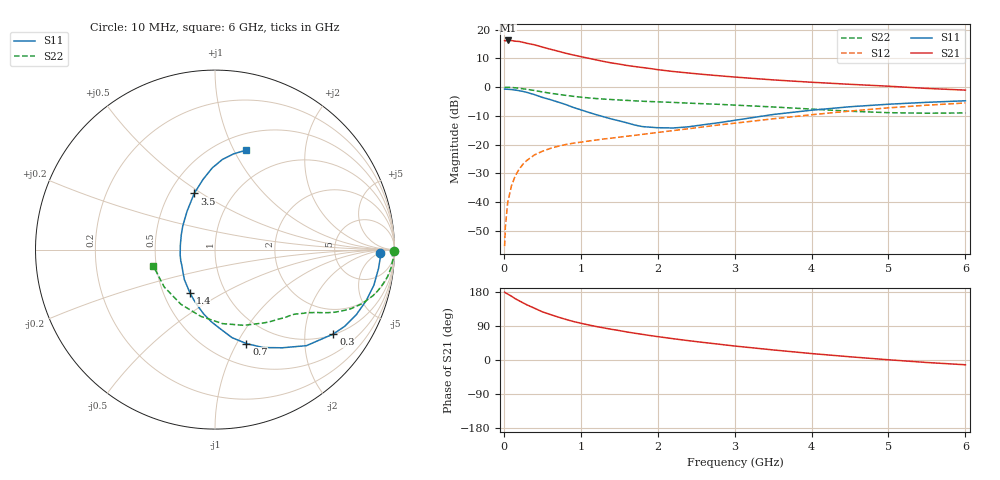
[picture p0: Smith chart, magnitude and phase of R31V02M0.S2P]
! SIEMENS Small Signal Semiconductors
! BFR181
! Si NPN RF Bipolar Junction Transistor in SOT23
! VCE = 1 V  IC = 2 mA
! Common Emitter S-Parameters:  May  1996
# GHz  S  MA  R  50
!  f  S11  S21  S12  S22
! GHz  MAG  ANG  MAG  ANG  MAG  ANG  MAG  ANG
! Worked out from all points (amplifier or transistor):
!   36 points, 10 MHz to 6 GHz, reference 50 ohm
!   highest |S21| = 16.3 dB at 50 MHz (marker M1)
!   |S21| within 3 dB of that: start of sweep to 597.3 MHz
!   unconditionally stable (mu >= 1): 1.503 GHz to 3.56 GHz
!   at 250 MHz: K = 0.24, MSG = 21.2 dB, |S12| = -26.8 dB
!   at 1.4 GHz: K = 0.97, MSG = 13.1 dB, |S12| = -17.8 dB
!   at 6 GHz: K = 0.89, MSG = 2.2 dB, |S12| = -5.5 dB
!   S11 on the Smith chart (normalised r, x): 10 MHz: 23, -6; 300 MHz: 1.02, -2.79; 700 MHz: 0.73, -1.10; 1.4 GHz: 0.68, -0.35; 3.5 GHz: 0.66, +0.47; 6 GHz: 0.67, +1.11
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0.01  0.922 -1.3  6.473 179.0  0.0017 93.9  0.9951 -0.6
0.02  0.9224 -2.5  6.391 177.4  0.0037 90.8  0.986 -1.2
0.05  0.9173 -6.5  6.498 174.1  0.0098 86.9  0.9934 -3.0
0.1  0.9071 -12.7  6.473 168.3  0.0193 82.5  0.9854 -6.0
0.15  0.889 -18.7  6.308 161.6  0.0288 77.8  0.9731 -8.9
0.2  0.8669 -24.7  6.236 156.2  0.0375 75.3  0.9558 -11.5
0.25  0.8402 -30.5  6.026 150.7  0.0457 71.8  0.9356 -14.2
0.3  0.8098 -35.5  5.797 145.5  0.053 69.5  0.9165 -16.3
0.4  0.739 -46.4  5.451 136.5  0.0663 64.4  0.8729 -20.2
0.5  0.663 -55.6  4.991 127.2  0.0762 60.3  0.826 -23.5
0.7  0.5521 -71.5  4.242 113.7  0.093 55.1  0.7511 -27.7
0.8  0.5001 -79.0  3.904 107.5  0.0999 53.0  0.7202 -29.2
0.9  0.4449 -85.8  3.635 101.8  0.1055 52.3  0.6928 -30.5
1.1  0.3641 -100.0  3.183 92.6  0.1151 51.0  0.6495 -32.7
1.4  0.2786 -120.2  2.637 81.0  0.1294 50.6  0.608 -35.7
1.7  0.219 -144.6  2.285 70.7  0.1445 51.6  0.577 -38.4
2.2  0.1944 173.6  1.873 56.2  0.1749 52.6  0.5419 -44.5
3  0.2643 126.1  1.498 36.9  0.2354 51.9  0.4864 -57.4
3.5  0.3336 110.3  1.337 26.6  0.2808 49.6  0.4516 -69.1
4.5  0.4555 91.9  1.12 8.5  0.3833 40.9  0.3801 -102.0
5.5  0.544 78.9  0.95 -6.6  0.4849 28.4  0.3512 -143.7
6  0.5788 72.9  0.887 -12.6  0.5297 21.1  0.3556 -165.1
